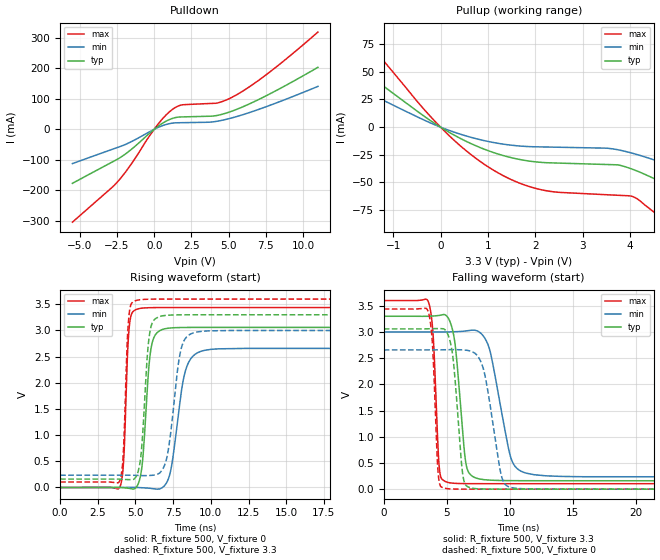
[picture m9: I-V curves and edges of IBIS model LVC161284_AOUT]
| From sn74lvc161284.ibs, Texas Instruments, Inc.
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[Model]   LVC161284_AOUT
Model_type  Output
Vref =   0
Rref =   500
Cref =   50p
Vmeas =   1.5
| variable   typ   min   max
C_comp   3.56pF   1.69pF   5.90pF
| C_pullup   3.41pF   2.14pF   4.10pF
| C_pulldown   3.71pF   1.69pF   5.90pF
[Temperature Range]   40   100   -40
| Ambient temperature   25   85   -40
[Voltage range]   3.3   3   3.6
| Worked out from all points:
|   slope of the pulldown table from 0 to 0.495 V, typ, clamps not added: 27.6 ohm
|   slope of the pullup table from 0 to 0.495 V, typ, clamps not added: 41.7 ohm
|   rising waveform, R_fixture 500, V_fixture 0: 20-80 % time 435ps typ, 765ps min, 261ps max; typ from 0 V to 3.06 V
|   falling waveform, R_fixture 500, V_fixture 3.3: 20-80 % time 667ps typ, 1.29ns min, 379ps max; typ from 3.3 V to 0.161 V
|   rising waveform, R_fixture 500, V_fixture 3.3: 20-80 % time 414ps typ, 676ps min, 257ps max; typ from 0.161 V to 3.3 V
|   falling waveform, R_fixture 500, V_fixture 0: 20-80 % time 607ps typ, 1.05ns min, 358ps max; typ from 3.06 V to 0 V
[Pulldown]
| LVC161284_AOUT
|   Voltage   I(typ)   I(min)   I(max)
-5.5V     -177.6mA   -112.8mA   -305.4mA
-2.435V   -97.24mA   -59.13mA   -170.9mA
-1.59V    -68.03mA   -41.88mA   -117.3mA
145mV     5.682mA    3.501mA    9.654mA
675mV     23.4mA     13.95mA    40.96mA
1.165V    34.8mA     19.84mA    63.26mA
1.885V    40.65mA    21.74mA    80.37mA
4.225V    45.57mA    26.46mA    86.19mA
5.335V    61.71mA    39.02mA    108.1mA
6.375V    83.05mA    54.66mA    139mA
7.64V     113.2mA    76.37mA    183.7mA
11V       203.7mA    141mA      319.5mA
[Pullup]
| LVC161284_AOUT
|   Voltage   I(typ)   I(min)   I(max)
-5.5V     174.8mA    117.5mA    276.7mA
-4.34V    138.3mA    92.57mA    219.8mA
-3.175V   100.9mA    67.07mA    161.1mA
-2.095V   65.8mA     43.4mA     105.8mA
-1.585V   49.29mA    32.33mA    79.56mA
1.12V     -23.01mA   -13.92mA   -38.98mA
2.225V    -32.11mA   -17.95mA   -57.43mA
4.04V     -37.88mA   -23.48mA   -62.54mA
4.9V      -55.04mA   -35.49mA   -90.5mA
6.405V    -91.99mA   -60.48mA   -150.2mA
8.23V     -140.1mA   -92.75mA   -228.5mA
11V       -214.9mA   -142.9mA   -350.8mA
[Ramp]
| LVC161284_AOUT
| variable   typ   min   max
dV/dt_r   1.85/4.48E-10   1.61/7.76E-10   2.08/2.74E-10
dV/dt_f   1.90/6.82E-10   1.68/1.30E-09   2.11/3.89E-10
R_load = 500
[Rising Waveform]
| LVC161284_AOUT
R_fixture =   500
C_fixture =   0
L_fixture =   0
V_fixture =   0
V_fixture_min = 0
V_fixture_max = 0
|   Time   V(typ)   V(min)   V(max)
0s        81.15pV    6.348nV    51.4pV
3.965ns   1.161mV    254.9uV    9.225mV
4.22ns    -4.222mV   611.9uV    555.8mV
4.595ns   -17.35mV   1.215mV    3.096V
5.205ns   87.87mV    -1.264mV   3.415V
6.03ns    2.655V     -17.86mV   3.436V
6.93ns    3.031V     34.84mV    3.438V
8.325ns   3.057V     2.24V      3.438V
9.595ns   3.058V     2.621V     3.438V
50ns      3.059V     2.658V     3.438V
[Falling Waveform]
| LVC161284_AOUT
R_fixture =   500
C_fixture =   0
L_fixture =   0
V_fixture =   3.3
V_fixture_min = 3
V_fixture_max = 3.6
|   Time   V(typ)   V(min)   V(max)
0s        3.3V       3V         3.6V
3.56ns    3.3V       2.999V     3.565V
3.94ns    3.305V     2.999V     2.869V
4.415ns   3.317V     2.999V     400.2mV
5.04ns    3.293V     3.001V     132.3mV
5.66ns    2.775V     3.005V     111.3mV
6.53ns    483mV      3.02V      105.8mV
7.415ns   205.6mV    3.021V     104.7mV
11.33ns   161.3mV    304.3mV    104.4mV
50ns      160.7mV    234.5mV    104.4mV
[Rising Waveform]
| LVC161284_AOUT
R_fixture =   500
C_fixture =   0
L_fixture =   0
V_fixture =   3.3
V_fixture_min = 3
V_fixture_max = 3.6
|   Time   V(typ)   V(min)   V(max)
0s        160.7mV    234.5mV    104.4mV
3.95ns    160.7mV    234.8mV    126.2mV
4.18ns    156.2mV    234.9mV    600.4mV
4.565ns   150.7mV    234.4mV    3.277V
5.105ns   247.9mV    231.1mV    3.577V
5.935ns   2.934V     229.2mV    3.598V
6.7ns     3.274V     306.9mV    3.6V
8.025ns   3.299V     2.645V     3.6V
9.02ns    3.3V       2.968V     3.6V
50ns      3.3V       3V         3.6V
[Falling Waveform]
| LVC161284_AOUT
R_fixture =   500
C_fixture =   0
L_fixture =   0
V_fixture =   0
V_fixture_min = 0
V_fixture_max = 0
|   Time   V(typ)   V(min)   V(max)
0s        3.059V     2.658V     3.438V
3.53ns    3.061V     2.657V     3.388V
3.865ns   3.063V     2.658V     2.777V
4.33ns    3.064V     2.659V     281.7mV
4.82ns    3.051V     2.66V      20.68mV
5.475ns   2.55V      2.663V     3.047mV
6.295ns   245.7mV    2.657V     505.1uV
6.885ns   26.37mV    2.635V     173.4uV
10.1ns    263.1uV    31.25mV    1.323uV
50ns      81.05pV    6.348nV    51.34pV
